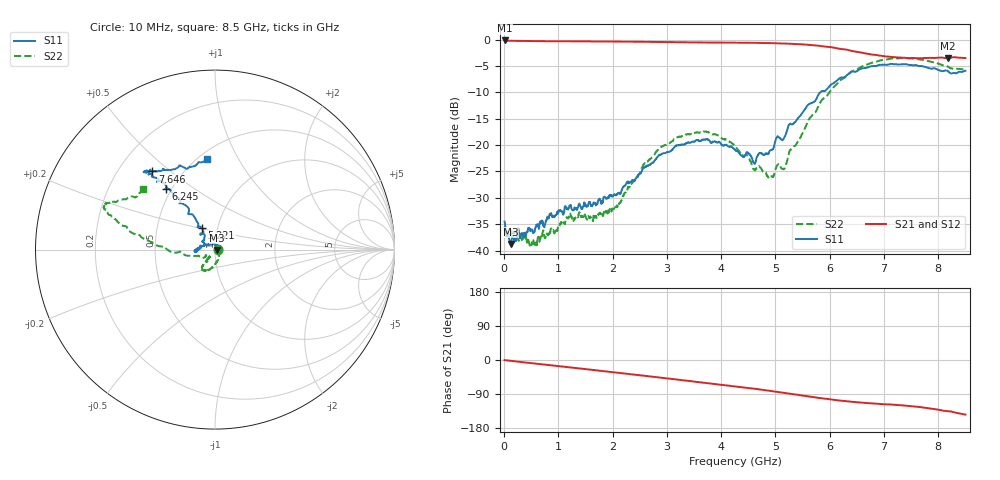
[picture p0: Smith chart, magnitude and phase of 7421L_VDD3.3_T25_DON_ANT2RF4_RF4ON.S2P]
!Agilent Technologies,E5071C,MY46417908,A.11.23
!Date: Thu Feb 25 16:17:30 2021
!Data & Calibration Information:
!Freq	S11:SOLT2(ON)	S21:SOLT2(ON)	S12:SOLT2(ON)	S22:SOLT2(ON)
!PortZ  Port1:50+j0  Port2:50+j0
!Above PortZ is port z conversion or system Z0 setting when saving the data.
!When reading, reference impedance value at option line is always used.
# Hz S dB R 50
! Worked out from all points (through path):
!   1601 points, 10 MHz to 8.5 GHz, reference 50 ohm
!   highest |S21| = -0.18 dB at 10 MHz (marker M1); lowest = -3.6 dB at 8.171 GHz (marker M2)
!   group delay of S21, straight-line fit = 46.6 ps
!   lowest |S11| = -38.7 dB at 126.7 MHz (marker M3), VSWR 1.02, Z = 51.2 - j0.165 ohm
!   |S11| at or under -10 dB: start of sweep to 5.827 GHz
!   |S22| runs from -39.2 to -3.5 dB; largest |S21 - S12| = 0.006
!   S11 on the Smith chart (normalised r, x): 10 MHz: 1.04, +0.00; 5.221 GHz: 0.84, +0.21; 6.245 GHz: 0.47, +0.39; 7.646 GHz: 0.34, +0.43; 8.5 GHz: 0.55, +0.75
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1e7  -34.50 2.4  -0.18 -0.4  -0.18 -0.4  -35.98 -7.3
1.267375e8  -38.73 -8.0  -0.24 -2.3  -0.25 -2.3  -36.83 -9.7
5.671562e8  -36.14 19.2  -0.31 -9.3  -0.31 -9.3  -38.70 22.2
1.182681e9  -32.11 44.4  -0.34 -19.1  -0.34 -19.1  -33.75 54.8
1.426769e9  -32.13 63.8  -0.36 -22.9  -0.36 -22.9  -33.51 45.5
1.644325e9  -31.12 71.4  -0.36 -26.4  -0.37 -26.4  -33.95 31.1
2.079438e9  -29.40 118.3  -0.40 -33.4  -0.40 -33.4  -31.43 -32.8
2.843538e9  -22.06 166.2  -0.47 -45.9  -0.47 -45.9  -20.81 -92.6
3.19375e9  -20.07 177.5  -0.51 -51.6  -0.51 -51.6  -18.54 -107.7
3.697844e9  -18.96 -176.1  -0.57 -60.0  -0.56 -60.1  -17.46 -122.3
4.255e9  -20.93 179.0  -0.60 -69.4  -0.60 -69.4  -20.13 -128.6
4.605212e9  -23.42 158.1  -0.63 -75.6  -0.62 -75.6  -24.61 -126.0
4.881138e9  -21.43 134.5  -0.68 -81.0  -0.67 -81.0  -26.00 -127.4
5.035019e9  -18.46 130.9  -0.73 -84.1  -0.72 -84.0  -23.79 -133.4
5.151756e9  -18.77 124.3  -0.76 -86.3  -0.76 -86.3  -24.60 -146.2
5.220738e9  -17.00 121.3  -0.78 -87.8  -0.78 -87.8  -22.81 -144.0
5.671769e9  -12.01 126.2  -1.08 -97.3  -1.06 -97.2  -14.41 -175.8
6.244844e9  -7.22 129.1  -1.84 -107.8  -1.85 -107.7  -7.41 169.2
7.088538e9  -4.72 131.2  -3.25 -117.1  -3.26 -117.4  -3.71 160.0
7.645694e9  -5.06 128.7  -3.55 -124.1  -3.58 -124.0  -3.77 156.4
8.171012e9  -5.95 112.2  -3.57 -135.1  -3.58 -135.4  -5.13 147.9
8.5e9  -5.91 95.2  -3.51 -144.0  -3.56 -144.3  -5.66 140.0
